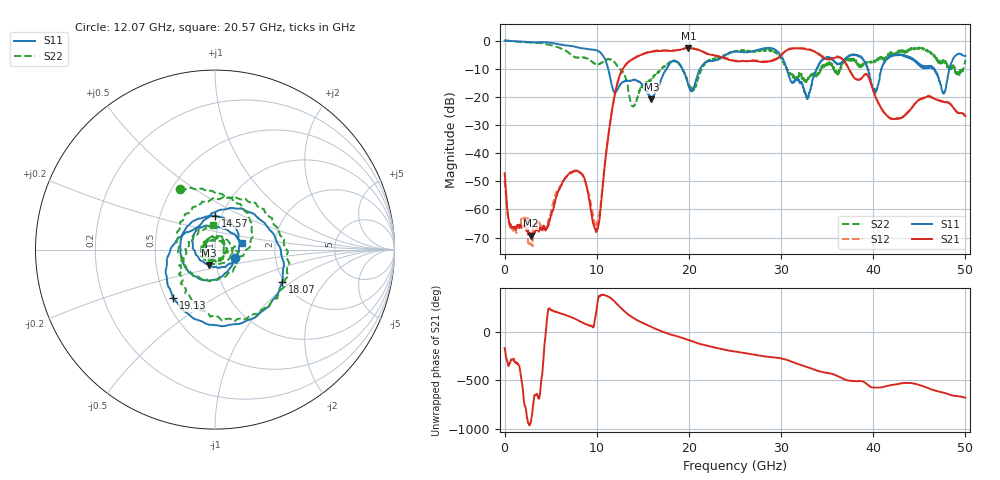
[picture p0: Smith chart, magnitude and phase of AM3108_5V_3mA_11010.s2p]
# Hz S DB R 50.0
!freq dBS11 angS11 dBS21 angS21 dBS12 angS12 dBS22 angS22
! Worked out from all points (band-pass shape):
!   1601 points, 10 MHz to 50 GHz, reference 50 ohm
!   highest |S21| = -2.62 dB at 19.94 GHz (marker M1); lowest = -69.3 dB at 2.822 GHz (marker M2)
!   |S21| within 3 dB of the highest: 14.46 GHz to 23.21 GHz (8.749 GHz wide, 46.5 % of centre); 29.9 GHz to 34.38 GHz (4.473 GHz wide, 13.9 % of centre)
!   lowest |S11| = -20.8 dB at 15.94 GHz (marker M3), VSWR 1.20, Z = 46.2 - j7.93 ohm
!   |S11| at or under -10 dB: 11.24 GHz to 17.6 GHz (6.351 GHz wide, 44 % of centre); 19.29 GHz to 21.22 GHz (1.935 GHz wide, 9.55 % of centre); 30.62 GHz to 33.85 GHz (3.227 GHz wide, 10 % of centre)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
!   |S22| runs from -23.4 to 0.0 dB; largest |S21 - S12| = 0.026
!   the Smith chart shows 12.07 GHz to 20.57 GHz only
!   S11 on the Smith chart (normalised r, x): 12.07 GHz: 1.25, -0.13; 14.57 GHz: 0.93, +0.37; 18.07 GHz: 1.95, -0.86; 19.13 GHz: 0.55, -0.34; 20.57 GHz: 1.35, +0.10
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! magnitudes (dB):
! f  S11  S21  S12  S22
! 10 MHz  0.0  -47.2  -49.8  0.0
! 666.1 MHz  -0.2  -65.5  -66.6  -0.2
! 2.26 GHz  -0.5  -66.2  -63.1  -0.6
! 2.822 GHz  -0.6  -69.3  -71.8  -0.7
! 8.352 GHz  -2.7  -47.3  -47.4  -5.9
! 10.07 GHz  -3.6  -66.7  -64.7  -8.6
! 12.07 GHz  -18.2  -17.6  -17.4  -8.2
! 13.88 GHz  -14.1  -6.6  -6.6  -23.4
! 14.57 GHz  -14.5  -5.4  -5.3  -18.9
! 15.94 GHz  -20.8  -4.0  -3.8  -13.8
! 16.69 GHz  -16.3  -3.8  -3.4  -11.4
! 18.07 GHz  -7.6  -3.7  -3.6  -7.2
! 19.13 GHz  -9.0  -3.2  -3.2  -9.2
! 19.94 GHz  -15.8  -2.6  -2.5  -15.9
! 20.57 GHz  -16.3  -3.0  -2.8  -17.2
! 25 GHz  -3.9  -7.3  -7.2  -3.9
! 33.35 GHz  -15.6  -3.5  -3.4  -12.7
! 38 GHz  -5.0  -13.5  -13.3  -6.6
! 40.22 GHz  -18.6  -19.8  -19.6  -7.6
! 41.69 GHz  -6.0  -27.3  -27.2  -5.3
! 47.66 GHz  -18.9  -21.8  -21.5  -7.7
! 50 GHz  -5.4  -26.9  -26.5  -6.9
